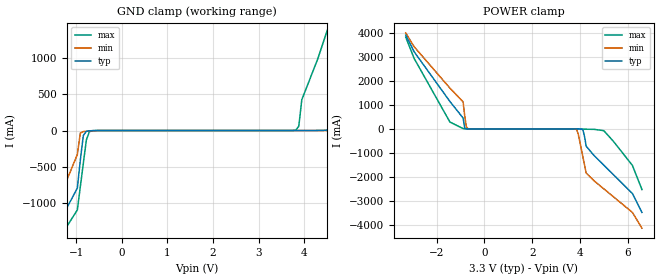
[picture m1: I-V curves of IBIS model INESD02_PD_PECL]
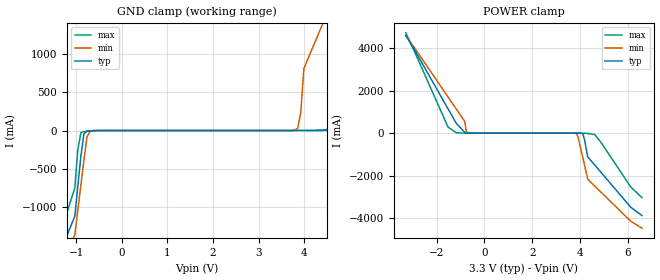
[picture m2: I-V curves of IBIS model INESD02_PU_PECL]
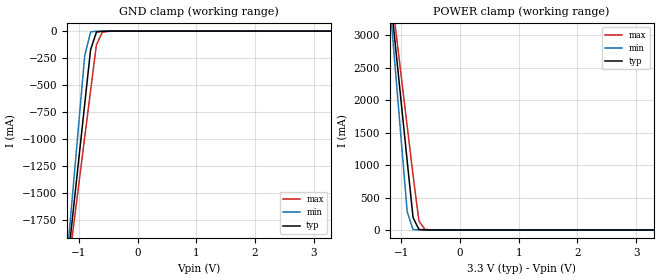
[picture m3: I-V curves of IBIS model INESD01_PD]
|   This file is an IBIS representation of the   |
|   Integrated Device Technology , Inc.   |
|   ICS8521I-03   |
|   Low Skew 1 to 9 Differential to LVHSTL Fanout Buffer   |
[IBIS Ver]   4.1
[File name]   8521i_03_3v3.ibs
[File Rev]   1.0
[Date]   16 Oct 2009 | Last modified
|   24 Aug 2000 | Generated
[Source]   Originated at Integrated Device Technology, Inc.
[Disclaimer]
IDT hereby grants the user of this IBIS model a non-exclusive,
nontransferable license to use this IBIS model under the following terms.
Before using this IBIS model, the user should read this license.
If the user does not accept these terms,  the IBIS model should be
returned to IDT within 30 days.
   The user is granted this license only to use the IBIS model and
is not granted rights to sell, load, rent, lease or license the IBIS
model in whole or in part, or in modified form to anyone other than
user. User may modify the IBIS model to suit its specific
applications but rights to derivative works and such modifications
shall belong to IDT.
   This IBIS model is provided on an "AS IS" basis and IDT makes
absolutely no warranty with respect to the information contained
herein. IDT DISCLAIMS AND CUSTOMER WAIVES ALL WARRANTIES, EXPRESS
OR IMPLIED, INCLUDING WARRANTIES OF MERCHANTABILITY OR FITNESS FOR
A PARTICULAR PURPOSE. The entire risk as to quality and performance
is with the Customer. ACCORDINGLY, IN NO EVENT SHALL THE COMPANY BE
LIABLE FOR ANY DAMAGES, WHETHER IN CONTRACT OR TORT,INCLUDING ANY
LOST PROFITS OR OTHER INCIDENTAL, CONSEQUENTIAL, EXEMPLARY, OR
PUNITIVE DAMAGES ARISING OUT OF THE USE OR APPLICATION OF THE IBIS
model provided in this package. Further, IDT reserves the right to
make changes without notice to any product herein to improve
reliability, function, or design. IDT does not convey any license
under patent rights or any other intellectual property rights,
including those of third parties.
   IDT is not obligated to provide maintenance or support
for the licensed IBIS model.
[Copyright]   Copyright 2005 by Integrated Device Technology , Inc.
[Component]   ICS8521YI-03
[Manufacturer] Integrated Device Technology, Inc.
[Package]
|LQFP32
|lead + wire   typ   min   max
R_pkg   220.4m   212.5m   238m
L_pkg   1.841n   1.708n   1.974n
C_pkg   0.316p   0.2907p   0.33p
[Pin] signal_name  model_name   R_pin   L_pin   C_pin
1   VDD   POWER   238m   1.974n   0.330p
2   CLK0   INESD02_PD_PECL   225m   1.841n   0.311p
3   nCLK0   INESD02_PU_PECL   218m   1.7745n   0.301p
4   CLK_SEL   INESD01_PD   213m   1.708n   0.291p
5   CLK1   INESD02_PD_PECL   213m   1.708n   0.291p
6   nCLK1   INESD02_PU_PECL   218m   1.7745n   0.301p
7   GND   GND   225m   1.841n   0.311p
8   CLK_EN   INESD01_PU   238m   1.974n   0.330p
9   VCCO   POWER   238m   1.974n   0.330p
10   nQ8   1v0_ONF01_HSTL01   225m   1.841n   0.311p
11   Q8   1v0_ONF01_HSTL01   218m   1.7745n   0.301p
12   nQ7   1v0_ONF01_HSTL01   213m   1.708n   0.291p
13   Q7   1v0_ONF01_HSTL01   213m   1.708n   0.291p
14   nQ6   1v0_ONF01_HSTL01   218m   1.7745n   0.301p
15   Q6   1v0_ONF01_HSTL01   225m   1.841n   0.311p
16   VDDO   POWER   238m   1.974n   0.330p
17   VDDO   POWER   238m   1.974n   0.330p
18   nQ5   1v0_ONF01_HSTL01   225m   1.841n   0.311p
19   Q5   1v0_ONF01_HSTL01   218m   1.7745n   0.301p
20   nQ4   1v0_ONF01_HSTL01   213m   1.708n   0.291p
21   Q4   1v0_ONF01_HSTL01   213m   1.708n   0.291p
22   nQ3   1v0_ONF01_HSTL01   218m   1.7745n   0.301p
23   Q3   1v0_ONF01_HSTL01   225m   1.841n   0.311p
24   VDDO   POWER   238m   1.974n   0.330p
25   VDDO   POWER   238m   1.974n   0.330p
26   nQ2   1v0_ONF01_HSTL01   225m   1.841n   0.311p
27   Q2   1v0_ONF01_HSTL01   218m   1.7745n   0.301p
28   nQ1   1v0_ONF01_HSTL01   213m   1.708n   0.291p
29   Q1   1v0_ONF01_HSTL01   213m   1.708n   0.291p
30   nQ0   1v0_ONF01_HSTL01   218m   1.7745n   0.301p
31   Q0   1v0_ONF01_HSTL01   225m   1.841n   0.311p
32   VDDO   POWER   238m   1.974n   0.330p
[Diff Pin]  inv_pin  vdiff tdelay_typ tdelay_min  tdelay_max
2   3   0.15   0   0   0
5   6   0.15   0   0   0
11   10   NA   0   0   0
13   12   NA   0   0   0
15   14   NA   0   0   0
19   18   NA   0   0   0
21   20   NA   0   0   0
23   22   NA   0   0   0
27   26   NA   0   0   0
29   28   NA   0   0   0
31   30   NA   0   0   0
| Models and submodels in the file (5): INESD02_PD_PECL (Input), INESD02_PU_PECL (Input), INESD01_PD (Input), INESD01_PU (Input), 1v0_ONF01_HSTL01 (Output_ECL)
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[Model]   INESD02_PD_PECL
Model_type  Input
Polarity   Non-Inverting
Vinl = 0.8V
Vinh = 2.0V
|   typ   min   max
C_comp   2pF   1.5pF   2.5pF
|   typ   min   max
[Voltage range]  3.3V   3.15V   3.45V
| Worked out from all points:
|   GND clamp passes 1 mA (typ) near -0.59 V on its own axis
|   POWER clamp passes 1 mA (typ) near -0.70 V on its own axis
[GND_clamp]
-3.3V     -3.894A    -4.294A    -3.674A
-1.6V     -1.569A    -1.322A    -1.74A
-974.8mV  -794.1mA   -331.5mA   -1.096A
-843.4mV  -68.33mA   -15.34mA   -452.9mA
-646.5mV  -1.912mA   -4.151mA   -2.665mA
3.818V    89.38uA    70.49uA    7.198mA
3.95V     342.2uA    75.94uA    423.8mA
4.6V      7.437mA    165.5uA    1.553A
4.9V      78.32mA    440.9uA    2.118A
5.5V      1.293A     2.769mA    3.249A
6.25V     2.651A     112.4mA    4.38A
6.6V      3.331A     896.1mA    4.946A
[POWER_clamp]
-3.3V     3.923A     4.017A     3.838A
-2.95V    3.23A      3.44A      2.951A
-1.45V    1.149A     1.709A     289.6mA
-896.9mV  456.5mA    1.133A     15.4mA
-762.9mV  4.223mA    91.07mA    1.486mA
-695.9mV  792.2uA    10.73mA    555.6uA
3.861V    -556.7uA   -26.14mA   -39.45uA
4.129V    -41.85mA   -1.19A     -4.904mA
4.263V    -724.2mA   -1.847A    -12.04mA
5V        -1.514A    -2.505A    -71.38mA
6.2V      -2.701A    -3.492A    -1.525A
6.6V      -3.492A    -4.151A    -2.536A
[Model]   INESD02_PU_PECL
Model_type  Input
Polarity   Non-Inverting
Vinl = 0.8V
Vinh = 2.0V
|   typ   min   max
C_comp   2pF   1.5pF   2.5pF
|   typ   min   max
[Voltage range]  3.3V   3.15V   3.45V
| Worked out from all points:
|   GND clamp passes 1 mA (typ) near -0.59 V on its own axis
|   POWER clamp passes 1 mA (typ) near -0.70 V on its own axis
[GND_clamp]
|Voltage   I(typ)   I(min)   I(max)
-3.3V     -3.894A    -3.674A    -4.294A
-1.3V     -1.521A    -1.7A      -1.261A
-1.031V   -1.125A    -1.372A    -755.3mA
-896.9mV  -335.4mA   -714.7mA   -27.07mA
-695.9mV  -3.401mA   -10.69mA   -6.477mA
3.794V    17.99uA    3.319mA    6.081uA
3.928V    181.1uA    239mA      10.12uA
3.995V    711.6uA    813.7mA    20.78uA
4.8V      40.44mA    1.967A     268.6uA
5.6V      1.139A     3.12A      2.243mA
6.3V      2.525A     4.275A     64.01mA
6.6V      3.219A     4.852A     752.7mA
[POWER_clamp]
|Voltage   I(typ)   I(min)   I(max)
-3.3V     4.617A     4.594A     4.726A
-1.53V    1.149A     1.709A     289.6mA
-1.18V    456.4mA    1.132A     15.33mA
-829.9mV  42.02mA    556.1mA    3.39mA
-762.9mV  4.159mA    91mA       1.422mA
-695.9mV  727.9uA    10.66mA    491.6uA
3.861V    -620.9uA   -26.2mA    -103.4uA
4.129V    -41.91mA   -1.19A     -4.968mA
4.33V     -1.119A    -2.176A    -17.93mA
4.63V     -1.515A    -2.505A    -71.45mA
6.13V     -3.492A    -4.151A    -2.536A
6.6V      -3.888A    -4.48A     -3.041A
[Model]   INESD01_PD
Model_type   Input
Polarity   Non-Inverting
Vinl = 0.80V
Vinh = 2.0V
|   typ   min   max
C_comp   2pF   1.5pF   2.5pF
|   typ   min   max
[Voltage range]  3.3V   3.15V   3.45V
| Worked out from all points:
|   GND clamp passes 1 mA (typ) near -0.55 V on its own axis
|   POWER clamp passes 1 mA (typ) near -0.60 V on its own axis
[GND_clamp]
|Voltage I(typ)   I(min)   I(max)
-3.3V     -12.83A    -15.14A    -11.37A
-1.2V     -2.195A    -2.092A    -2.281A
-1.1V     -1.689A    -1.472A    -1.849A
-900mV    -678.5mA   -232.6mA   -984.8mA
-800mV    -173.9mA   -7.175mA   -553.2mA
-700mV    -9.696mA   -1.052mA   -126mA
-600mV    -1.629mA   -178uA     -11.07mA
-300mV    -10.53uA   -5.678uA   -86.08uA
3.3V      71.13uA    62.11uA    77.58uA
[POWER_clamp]
|Voltage   I(typ)   I(min)   I(max)
-3.3V     22.38A     26.45A     19.82A
-1.2V     3.723A     3.545A     3.874A
-1.1V     2.836A     2.457A     3.116A
-1V       1.949A     1.369A     2.358A
-900mV    1.063A     281.1mA    1.601A
-800mV    191.6mA    5.074mA    844mA
-700mV    8.104mA    204.3uA    138.4mA
-600mV    678.1uA    79.74uA    10.7mA
-400mV    87.44uA    69.65uA    413.2uA
3.3V      -3.041nA   -425fA     -919.9nA
